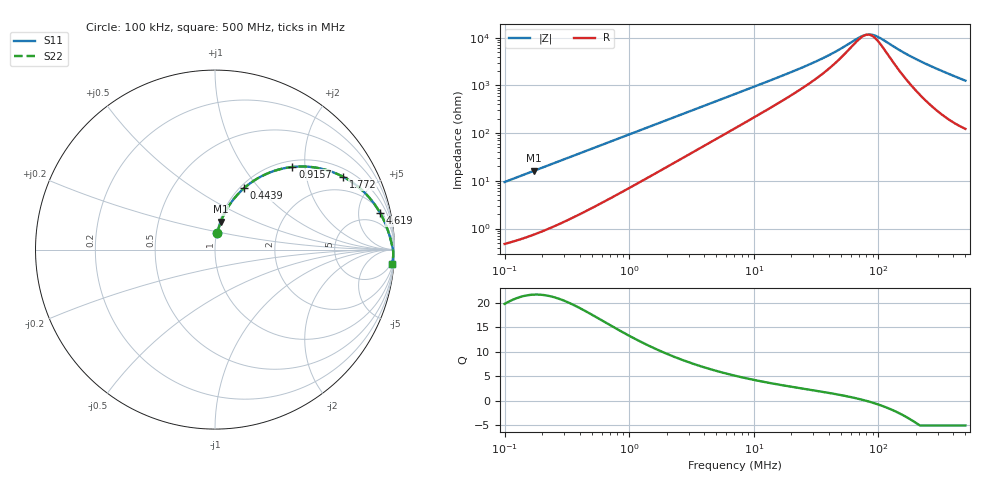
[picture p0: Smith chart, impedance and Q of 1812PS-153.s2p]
# MHz S MA R 50
!Freq  MagS11  AngS11  MagS21  AngS21  MagS12  AngS12  MagS22  AngS22
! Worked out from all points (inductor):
!   801 points, 100 kHz to 500 MHz, reference 50 ohm
!   read as one part in series: L = 15 uH near 104.4 kHz
!   highest Q = 21.7 at 172.1 kHz (marker M1), where L = 15 uH
!   self-resonance near 80.59 MHz
!   S11 on the Smith chart (normalised r, x): 100 kHz: 1.01, +0.19; 443.9 kHz: 1.05, +0.83; 915.7 kHz: 1.12, +1.72; 1.772 MHz: 1.32, +3.31; 4.619 MHz: 2.34, +8.53; 500 MHz: 3, -25
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0.1  0.09346 81.7  0.9909 -5.4  0.9909 -5.4  0.09346 81.7
0.1721113  0.159 78.2  0.98 -9.1  0.98 -9.1  0.159 78.2
0.2778922  0.2504 72.8  0.9562 -14.5  0.9562 -14.5  0.2504 72.8
0.416464  0.3587 66.0  0.9145 -21.0  0.9145 -21.0  0.3587 66.0
0.4439354  0.3784 64.7  0.9052 -22.2  0.9052 -22.2  0.3784 64.7
0.624135  0.4934 57.0  0.8399 -29.5  0.8399 -29.5  0.4934 57.0
0.9156557  0.6304 46.9  0.732 -39.0  0.732 -39.0  0.6304 46.9
1.233662  0.7281 38.7  0.628 -46.5  0.628 -46.5  0.7281 38.7
1.716055  0.8152 30.2  0.506 -54.2  0.506 -54.2  0.8152 30.2
1.77175  0.8223 29.5  0.4944 -54.9  0.4944 -54.9  0.8223 29.5
2.770756  0.8975 20.1  0.3457 -63.0  0.3457 -63.0  0.8975 20.1
4.618878  0.9426 12.5  0.2184 -68.6  0.2184 -68.6  0.9426 12.5
7.071068  0.9618 8.2  0.1459 -70.8  0.1459 -70.8  0.9618 8.2
29.44845  0.9855 1.8  0.0338 -63.8  0.0338 -63.8  0.9855 1.8
42.29302  0.9881 1.0  0.02145 -55.8  0.02145 -55.8  0.9881 1.0
69.01754  0.9907 0.2  0.01011 -23.5  0.01011 -23.5  0.9907 0.2
78.4231  0.9913 0.0  0.008745 -4.6  0.008745 -4.6  0.9913 0.0
85.39525  0.9916 -0.1  0.008515 10.1  0.008515 10.1  0.9916 -0.1
93.98253  0.992 -0.2  0.008978 26.4  0.008978 26.4  0.992 -0.2
121.3434  0.9928 -0.6  0.01314 56.2  0.01314 56.2  0.9928 -0.6
220.2643  0.9935 -1.8  0.03152 77.3  0.03152 77.3  0.9935 -1.8
500  0.9892 -4.5  0.07885 79.9  0.07885 79.9  0.9892 -4.5
